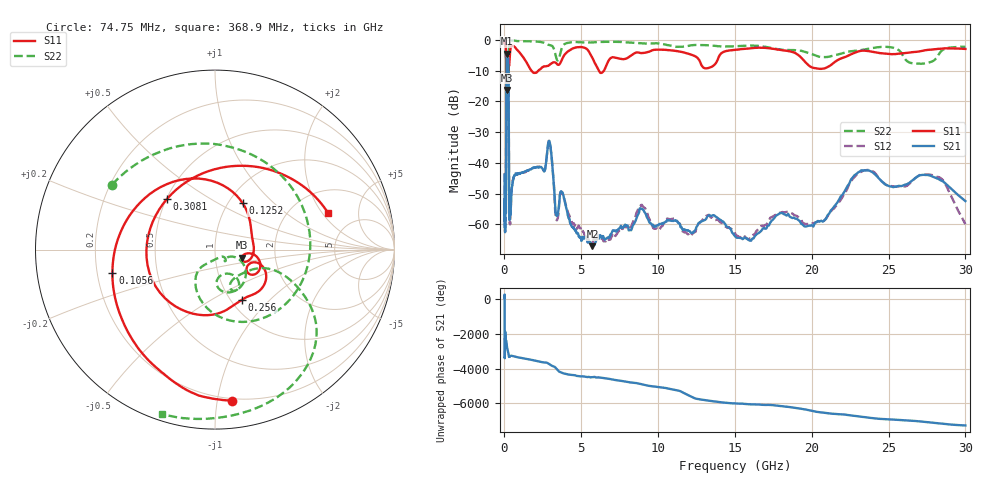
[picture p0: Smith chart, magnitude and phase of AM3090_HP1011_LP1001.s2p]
! Date/Time: Thu, Feb 28, 2019 2:05 PM
! Network Analyzer: Agilent Technologies E8364B Rev: A.07.50.67
! Sweep from 0.010 to 30.000 GHz, 1601 Points, Sweep Type: LOG
! Power Supply: 5.023 V, 0.002 A
# Hz S DB R 50
!freq MagS11 AngS11 MagS21 AngS21 MagS12 AngS12 MagS22 AngS22
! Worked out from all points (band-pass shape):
!   1601 points, 10 MHz to 30 GHz, reference 50 ohm
!   highest |S21| = -4.38 dB at 171.5 MHz (marker M1); lowest = -67.2 dB at 5.725 GHz (marker M2)
!   |S21| within 3 dB of the highest: 131 MHz to 253.7 MHz (122.6 MHz wide, 63.8 % of centre)
!   lowest |S11| = -16.2 dB at 158.3 MHz (marker M3), VSWR 1.37, Z = 67.1 - j6.07 ohm
!   |S11| at or under -10 dB: 124.4 MHz to 230 MHz (105.7 MHz wide, 59.6 % of centre); 1.762 GHz to 2.203 GHz (440.7 MHz wide, 22.2 % of centre); 6.147 GHz to 6.467 GHz (320.8 MHz wide, 5.09 % of centre)
!   |S22| runs from -26.1 to -0.1 dB; largest |S21 - S12| = 0.013
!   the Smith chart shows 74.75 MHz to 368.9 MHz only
!   S11 on the Smith chart (normalised r, x): 74.75 MHz: 0.18, -1.10; 105.6 MHz: 0.26, -0.10; 125.2 MHz: 1.16, +0.66; 256 MHz: 1.13, -0.70; 308.1 MHz: 0.50, +0.34; 368.9 MHz: 3.17, +2.29
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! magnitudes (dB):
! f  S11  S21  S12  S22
! 10 MHz  -0.3  -43.9  -43.4  -0.7
! 38.04 MHz  -0.4  -60.1  -59.1  -1.5
! 74.75 MHz  -1.4  -53.3  -53.6  -3.4
! 95.52 MHz  -3.3  -55.6  -52.0  -5.1
! 105.6 MHz  -4.6  -38.0  -38.0  -5.5
! 125.2 MHz  -10.4  -10.6  -10.6  -16.3
! 144.7 MHz  -13.7  -5.2  -5.2  -21.6
! 158.3 MHz  -16.2  -4.5  -4.5  -19.5
! 171.5 MHz  -13.4  -4.4  -4.3  -13.7
! 256 MHz  -10.0  -7.8  -7.7  -14.2
! 308.1 MHz  -8.2  -55.6  -54.1  -1.0
! 368.9 MHz  -3.6  -56.9  -59.9  -0.3
! 550.5 MHz  -2.0  -45.9  -45.8  -0.2
! 2.084 GHz  -10.6  -41.4  -41.4  -0.5
! 2.928 GHz  -8.1  -33.0  -33.1  -1.6
! 3.402 GHz  -7.7  -57.3  -58.7  -6.3
! 3.76 GHz  -6.1  -49.6  -50.1  -2.3
! 5.725 GHz  -5.8  -67.2  -66.1  -0.8
! 7.926 GHz  -6.0  -60.5  -61.0  -0.7
! 15.81 GHz  -2.8  -64.7  -64.9  -1.8
! 23.48 GHz  -3.5  -42.4  -42.5  -3.0
! 30 GHz  -2.9  -52.5  -60.0  -2.2
